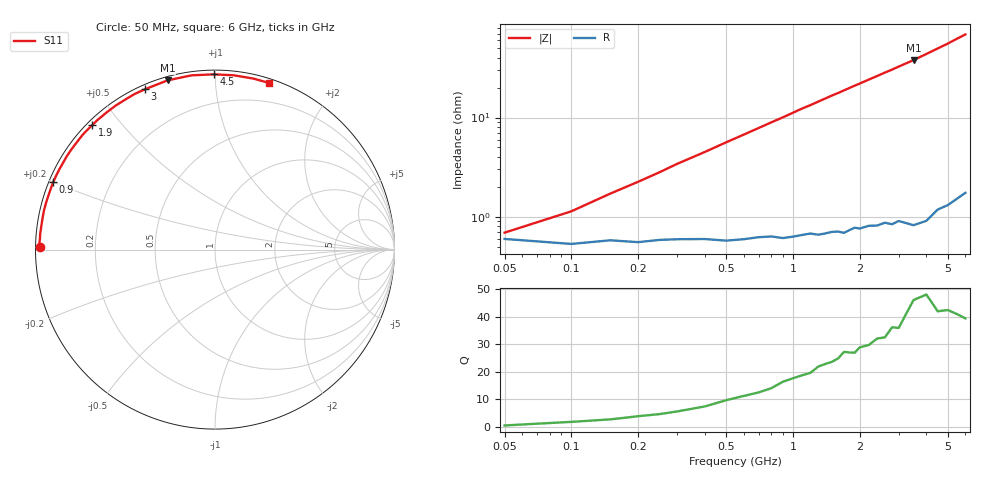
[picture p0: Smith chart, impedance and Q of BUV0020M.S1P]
! Infineon Technologies  Discrete & RF Semiconductors
! BB 833
! Si Tuning Diode in SOD323
! VR =
! S-Parameters:  June  1999
# GHz  S  MA  R  50
!  f  S11
! GHz  MAG  ANG
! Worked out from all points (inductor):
!   34 points, 50 MHz to 6 GHz, reference 50 ohm
!   read as one part to ground: L = 1.75 nH near 200 MHz
!   highest Q = 46 at 3.5 GHz (marker M1), where L = 1.73 nH
!   S11 on the Smith chart (normalised r, x): 50 MHz: 0.01, +0.01; 900 MHz: 0.01, +0.20; 1.9 GHz: 0.02, +0.42; 3 GHz: 0.02, +0.65; 4.5 GHz: 0.02, +0.99; 6 GHz: 0.03, +1.38
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0.05  0.9763 179.2
0.1  0.9789 177.7
0.15  0.9771 176.3
0.2  0.9781 175.0
0.3  0.9766 172.3
0.5  0.9775 167.2
0.6  0.9769 164.7
0.8  0.9757 159.7
0.9  0.9768 157.3
1.1  0.9755 152.3
1.2  0.975 150.1
1.3  0.9759 147.7
1.5  0.9749 143.1
1.6  0.975 141.0
1.7  0.9761 138.8
1.9  0.9739 134.5
2  0.9748 132.5
2.2  0.974 128.4
2.4  0.9747 124.6
2.6  0.9739 120.8
2.8  0.9757 117.3
3  0.9748 113.7
3.5  0.9793 105.6
4  0.9796 97.6
4.5  0.9765 90.3
5  0.9768 83.8
5.5  0.9765 77.4
6  0.9761 72.0
